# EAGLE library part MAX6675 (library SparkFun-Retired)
Cold-Junction-Compensated K-Thermocoupleto-Digital Converter (0°C to +1024°C) The MAX6675 performs cold-junction compensation and digitizes the signal from a type-K thermocouple. The data is output in a 12-bit resolution, SPI™-compatible, read-only format. This converter resolves temperatures to 0.25°C, allows readings as high as +1024°C, and exhibits thermocouple accuracy of 8LSBs for temperatures ranging from 0°C to +700°C. Dead Prototype: IC-12512<br.
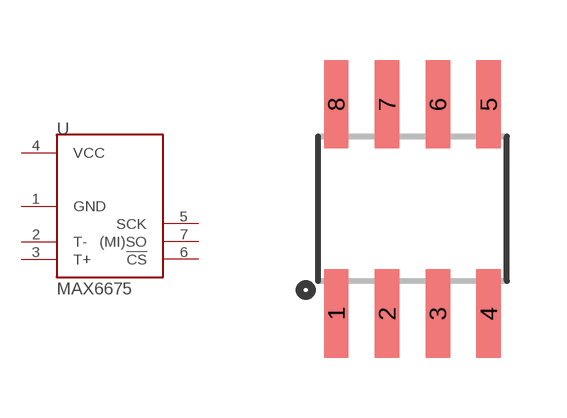
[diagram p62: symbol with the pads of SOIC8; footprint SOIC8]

Designator prefix U

## MAX6675 (PROD_ID: IC-12512)  [SOIC8]
1  GND
2  T-
3  T+
4  VCC
5  SCK
6  !CS
7  (MI)SO

## Footprint SOIC8 (pad centres in mm)
smd 0.61 x 2.21: 1 -1.905,-2.616; 2 -0.635,-2.616; 3 0.635,-2.616; 4 1.905,-2.616; 5 1.905,2.616; 6 0.635,2.616; 7 -0.635,2.616; 8 -1.905,2.616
